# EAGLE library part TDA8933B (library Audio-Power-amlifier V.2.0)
The TDA8933B is a high-efficiency class D amplifier with low power dissipation. The continuous time output power is 2 ´ 10 W in a stereo half-bridge application (RL = 8 W) or 1 ´ 20 W in a mono full-bridge application (RL =16 W). Due to the low power dissipation the device can be used without any external heat sink when playing music. Due to the implementation of Thermal Foldback (TF) the device remains operating with considerable music output power without the need for an external heat sink, even for high supply voltages and/or lower load impedances.
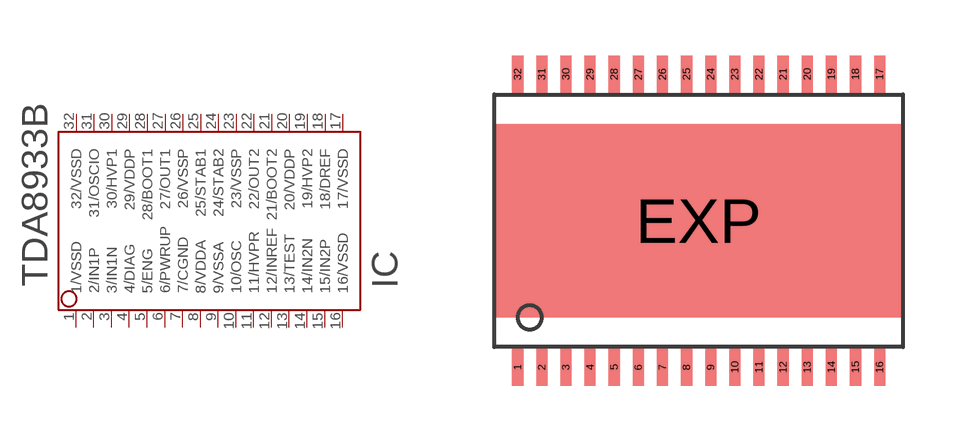
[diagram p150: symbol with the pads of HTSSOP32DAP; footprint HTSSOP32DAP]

Designator prefix IC

## TDA8933B  [HTSSOP32DAP]
1  1/VSSD  pwr
2  2/IN1P  in
3  3/IN1N  in
4  4/DIAG  out
5  5/ENG  in
6  6/PWRUP  in
7  7/CGND  pwr
8  8/VDDA  pwr
9  9/VSSA  pwr
10  10/OSC  in
11  11/HVPR  pwr
12  12/INREF  in
13  13/TEST  in
14  14/IN2N  in
15  15/IN2P  in
16  16/VSSD  pwr
17  17/VSSD  pwr
18  18/DREF
19  19/HVP2  out
20  20/VDDP  pwr
21  21/BOOT2
22  22/OUT2  out
23  23/VSSP  out
24  24/STAB2
25  25/STAB1
26  26/VSSP  pwr
27  27/OUT1  out
28  28/BOOT1
29  29/VDDP  pwr
30  30/HVP1
31  31/OSCIO  in
32  32/VSSD  pwr

## Footprint HTSSOP32DAP (pad centres in mm)
PowerPAD(TM) PLASTIC SMALL-OUTLINE PACKAGE
smd 0.3 x 1: 1 -4.875,-3.95; 2 -4.225,-3.95; 3 -3.575,-3.95; 4 -2.925,-3.95; 5 -2.275,-3.95; 6 -1.625,-3.95; 7 -0.975,-3.95; 8 -0.325,-3.95; 9 0.325,-3.95; 10 0.975,-3.95; 11 1.625,-3.95; 12 2.275,-3.95; 13 2.925,-3.95; 14 3.575,-3.95; 15 4.225,-3.95; 16 4.875,-3.95; 17 4.875,3.95; 18 4.225,3.95; 19 3.575,3.95; 20 2.925,3.95; 21 2.275,3.95; 22 1.625,3.95; 23 0.975,3.95; 24 0.325,3.95; 25 -0.325,3.95; 26 -0.975,3.95; 27 -1.625,3.95; 28 -2.275,3.95; 29 -2.925,3.95; 30 -3.575,3.95; 31 -4.225,3.95; 32 -4.875,3.95
smd 11 x 5.2: EXP 0,0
